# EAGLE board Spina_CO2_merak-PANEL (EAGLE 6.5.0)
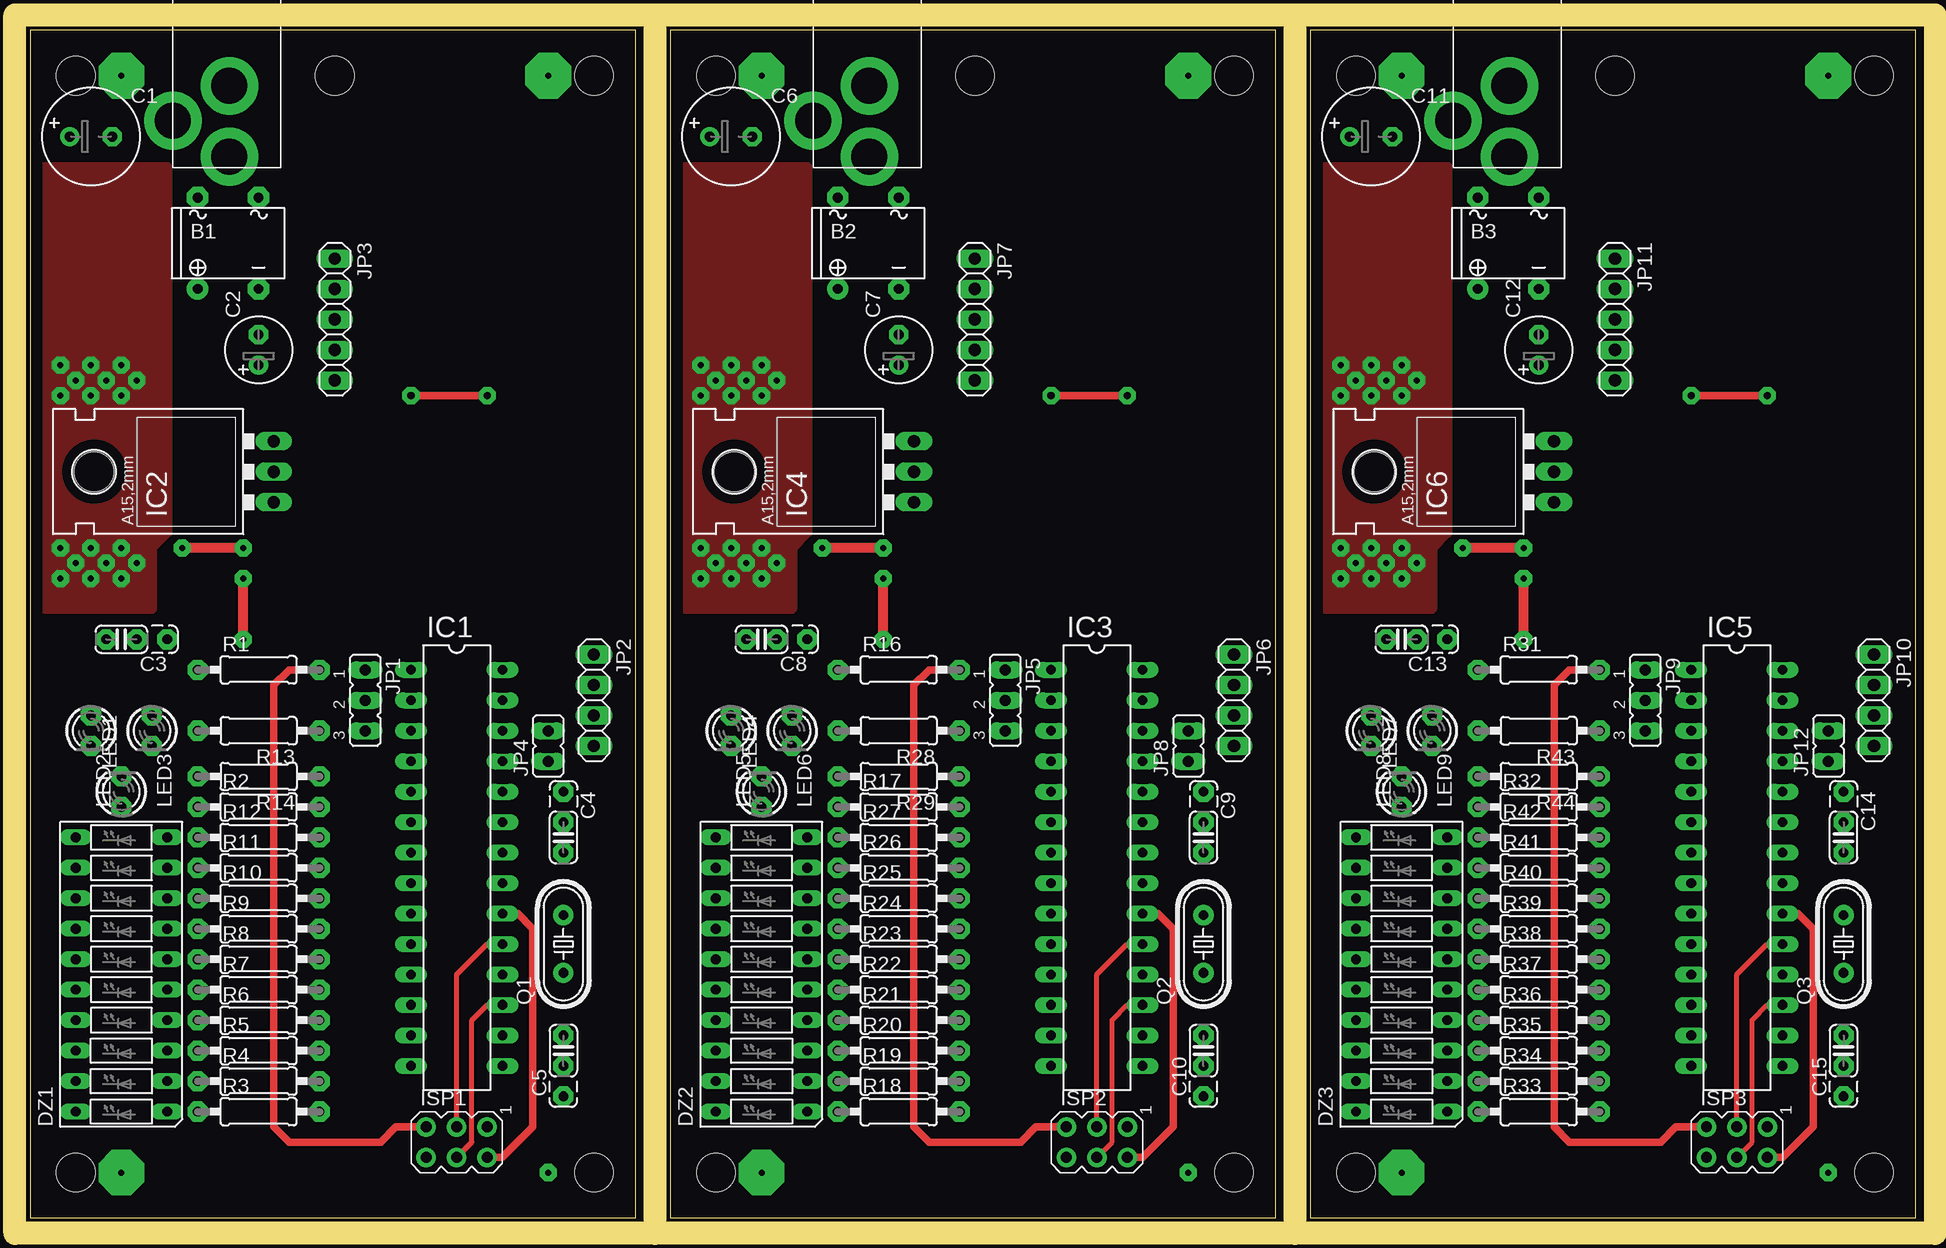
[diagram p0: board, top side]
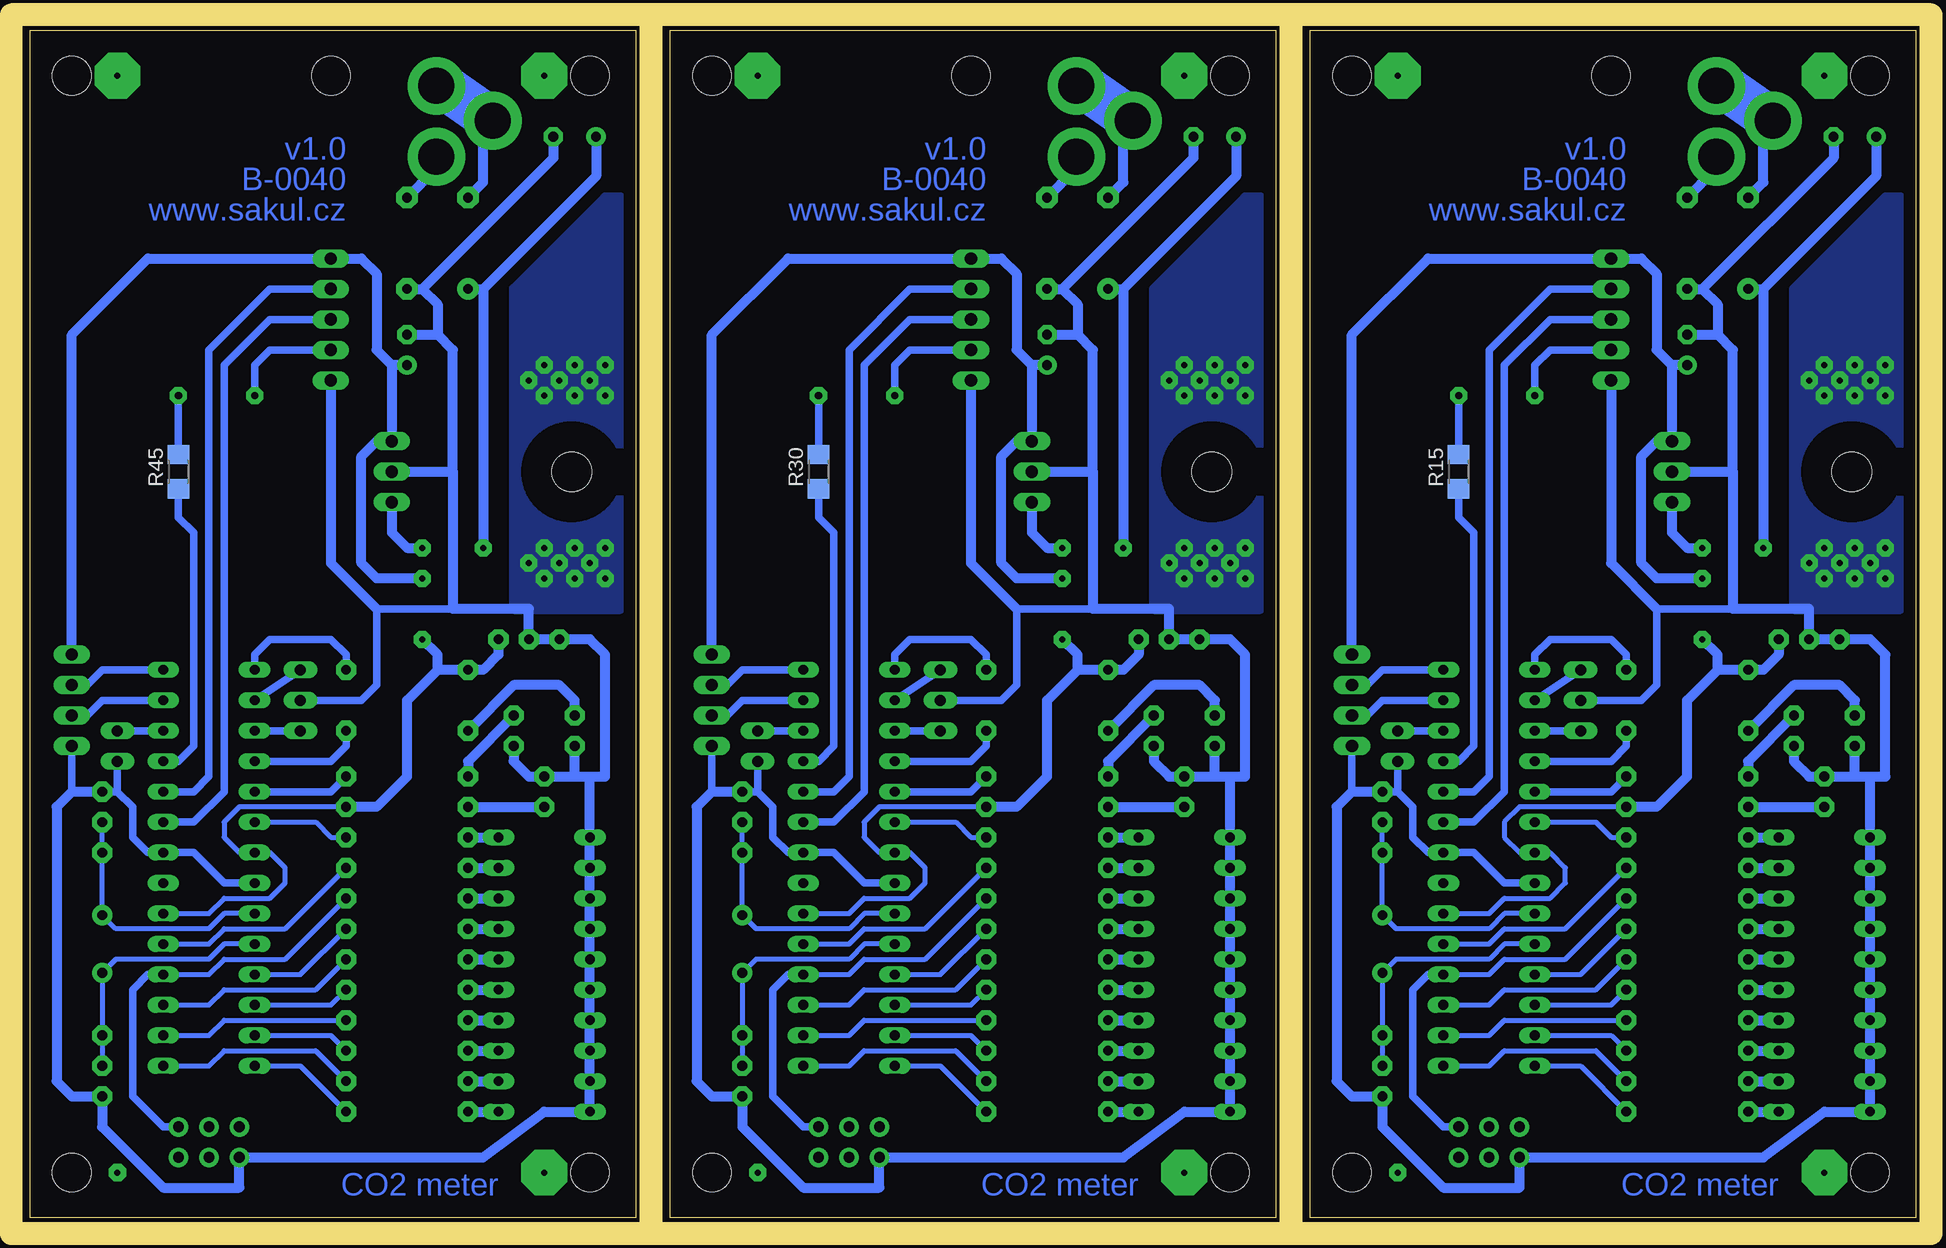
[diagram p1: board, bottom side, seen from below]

Size 157.15 x 99.04 mm. Coordinates in mm from the lower left corner, seen from the top.
Outline: 0,99.04 0,0 50.47,0 50.47,99.04 0,99.04
Outline: 53.34,99.04 53.34,0 103.81,0 103.81,99.04 53.34,99.04
Outline: 106.68,99.04 106.68,0 157.15,0 157.15,99.04 106.68,99.04
Copper layers (1*16): Top 0.035mm / dielectric 1.5mm / Bottom 0.035mm
Design rules "default": minimum track width 10mil, minimum drill 24mil, track to track 8mil, track to pad 8mil, pad to pad 8mil, via to via 8mil, smd to smd 8mil, copper to edge 40mil, drill to drill 8mil, minimum pad ring 10mil, minimum via ring 8mil, stop-mask expansion 4mil, vias tented up to drill 0mil, thermal gap 10mil
Holes 3.2 mm at 3.81,95.23 3.81,3.79 46.99,3.79 46.99,95.23 25.4,95.23 57.15,95.23 57.15,3.79 100.33,3.79 100.33,95.23 78.74,95.23 110.49,95.23 110.49,3.79 153.67,3.79 153.67,95.23 132.08,95.23
Milling: 10 lines

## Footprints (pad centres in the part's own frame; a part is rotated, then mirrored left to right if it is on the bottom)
B-DIL = drill 0.813 pad 1.778: + -2.54,-3.81 | drill 0.813 pad 1.778 octagon: - 2.54,-3.81; AC1 2.54,3.81; AC2 -2.54,3.81
E3,5-8 = drill 0.813 pad 1.6: + -1.778,0 | drill 0.813 pad 1.6 octagon: - 1.778,0
E2,5-6 = drill 0.813 pad 1.6: + -1.27,0 | drill 0.813 pad 1.6 octagon: - 1.27,0
C025_050-024X070 = drill 0.813 pad 1.676 octagon: 1 -3.81,0; 2 -1.27,0; 3 1.27,0
LB10 = drill 0.813 long: 1 -11.43,-3.81; 2 -8.89,-3.81; 3 -6.35,-3.81; 4 -3.81,-3.81; 5 -1.27,-3.81; 6 1.27,-3.81; 7 3.81,-3.81; 8 6.35,-3.81; 9 8.89,-3.81; 10 11.43,-3.81; 11 11.43,3.81; 12 8.89,3.81; 13 6.35,3.81; 14 3.81,3.81; 15 1.27,3.81; 16 -1.27,3.81; 17 -3.81,3.81; 18 -6.35,3.81; 19 -8.89,3.81; 20 -11.43,3.81
DIL28-3 = drill 0.813 long: 1 -16.51,-3.81; 2 -13.97,-3.81; 3 -11.43,-3.81; 4 -8.89,-3.81; 5 -6.35,-3.81; 6 -3.81,-3.81; 7 -1.27,-3.81; 8 1.27,-3.81; 9 3.81,-3.81; 10 6.35,-3.81; 11 8.89,-3.81; 12 11.43,-3.81; 13 13.97,-3.81; 14 16.51,-3.81; 15 16.51,3.81; 16 13.97,3.81; 17 11.43,3.81; 18 8.89,3.81; 19 6.35,3.81; 20 3.81,3.81; 21 1.27,3.81; 22 -1.27,3.81; 23 -3.81,3.81; 24 -6.35,3.81; 25 -8.89,3.81; 26 -11.43,3.81; 27 -13.97,3.81; 28 -16.51,3.81
78XXL = drill 1.016 long: GND 0,-3.81; IN -2.54,-3.81; OUT 2.54,-3.81 | hole 3.302: 0,11.176
AVRISP = drill 0.9 pad 1.626: 1 -1.27,2.54; 2 1.27,2.54; 3 -1.27,0; 4 1.27,0; 5 -1.27,-2.54; 6 1.27,-2.54
JP2 = drill 0.914 long: 1 -2.54,0; 2 0,0; 3 2.54,0
1X04 = drill 1.016 long: 1 -3.81,0; 2 -1.27,0; 3 1.27,0; 4 3.81,0
1X05 = drill 1.016 long: 1 -5.08,0; 2 -2.54,0; 3 0,0; 4 2.54,0; 5 5.08,0
JP1 = drill 0.914 long: 1 0,-1.27; 2 0,1.27
LED3MM = drill 0.813 pad 1.676 octagon: A -1.27,0; K 1.27,0
HC49/S = drill 0.813 pad 1.676: 1 -2.413,0; 2 2.413,0
0207/10 = drill 0.813 pad 1.676 octagon: 1 -5.08,0; 2 5.08,0
R1206 = smd 1.6 x 1.803: 1 -1.422,0; 2 1.422,0
PJ-102A = drill 3 pad 4.8: RING 0.1,-3.39; RING_SW -4.6,-6.29; TIP 0.1,-9.29

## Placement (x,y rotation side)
B1  [B-DIL]  16.51,81.26 0 top
B2  [B-DIL]  69.85,81.26 0 top
B3  [B-DIL]  123.19,81.26 0 top
C1  470uF/25V  [E3,5-8]  5.08,90.15 0 top
C2  100uF/10V  [E2,5-6]  19.05,72.37 90 top
C3  100nF  [C025_050-024X070]  7.62,48.24 180 top
C4  22pF  [C025_050-024X070]  44.45,31.73 270 top
C5  22pF  [C025_050-024X070]  44.45,13.95 90 top
C6  470uF/25V  [E3,5-8]  58.42,90.15 0 top
C7  100uF/10V  [E2,5-6]  72.39,72.37 90 top
C8  100nF  [C025_050-024X070]  60.96,48.24 180 top
C9  22pF  [C025_050-024X070]  97.79,31.73 270 top
C10  22pF  [C025_050-024X070]  97.79,13.95 90 top
C11  470uF/25V  [E3,5-8]  111.76,90.15 0 top
C12  100uF/10V  [E2,5-6]  125.73,72.37 90 top
C13  100nF  [C025_050-024X070]  114.3,48.24 180 top
C14  22pF  [C025_050-024X070]  151.13,31.73 270 top
C15  22pF  [C025_050-024X070]  151.13,13.95 90 top
DZ1  LB10  [LB10]  7.62,20.3 90 top
DZ2  LB10  [LB10]  60.96,20.3 90 top
DZ3  LB10  [LB10]  114.3,20.3 90 top
IC1  ATMEGA8-PU  [DIL28-3]  35.56,29.19 270 top
IC2  7805  [78XXL]  16.51,62.21 90 top
IC3  ATMEGA8-PU  [DIL28-3]  88.9,29.19 270 top
IC4  7805  [78XXL]  69.85,62.21 90 top
IC5  ATMEGA8-PU  [DIL28-3]  142.24,29.19 270 top
IC6  7805  [78XXL]  123.19,62.21 90 top
ISP1  AVRISP-6  [AVRISP]  35.56,6.33 270 top
ISP2  AVRISP-6  [AVRISP]  88.9,6.33 270 top
ISP3  AVRISP-6  [AVRISP]  142.24,6.33 270 top
JP1  [JP2]  27.94,43.16 270 top
JP2  [1X04]  46.99,43.16 270 top
JP3  [1X05]  25.4,74.91 270 top
JP4  [JP1]  43.18,39.35 0 top
JP5  [JP2]  81.28,43.16 270 top
JP6  [1X04]  100.33,43.16 270 top
JP7  [1X05]  78.74,74.91 270 top
JP8  [JP1]  96.52,39.35 0 top
JP9  [JP2]  134.62,43.16 270 top
JP10  [1X04]  153.67,43.16 270 top
JP11  [1X05]  132.08,74.91 270 top
JP12  [JP1]  149.86,39.35 0 top
LED1  [LED3MM]  7.62,35.54 90 top
LED2  [LED3MM]  5.08,40.62 270 top
LED3  [LED3MM]  10.16,40.62 270 top
LED4  [LED3MM]  60.96,35.54 90 top
LED5  [LED3MM]  58.42,40.62 270 top
LED6  [LED3MM]  63.5,40.62 270 top
LED7  [LED3MM]  114.3,35.54 90 top
LED8  [LED3MM]  111.76,40.62 270 top
LED9  [LED3MM]  116.84,40.62 270 top
Q1  16MHz  [HC49/S]  44.45,22.84 90 top
Q2  16MHz  [HC49/S]  97.79,22.84 90 top
Q3  16MHz  [HC49/S]  151.13,22.84 90 top
R1  12K  [0207/10]  19.05,45.7 0 top
R2  1K  [0207/10]  19.05,34.27 0 top
R3  1K  [0207/10]  19.05,8.87 0 top
R4  1K  [0207/10]  19.05,11.41 0 top
R5  1K  [0207/10]  19.05,13.95 0 top
R6  1K  [0207/10]  19.05,16.49 0 top
R7  1K  [0207/10]  19.05,19.03 0 top
R8  1K  [0207/10]  19.05,21.57 0 top
R9  1K  [0207/10]  19.05,24.11 0 top
R10  1K  [0207/10]  19.05,26.65 0 top
R11  1K  [0207/10]  19.05,29.19 0 top
R12  1K  [0207/10]  19.05,31.73 0 top
R13  1K  [0207/10]  19.05,40.62 180 top
R14  1K  [0207/10]  19.05,36.81 180 top
R15  NONE/0R  [R1206]  38.1,62.21 90 bottom
R16  12K  [0207/10]  72.39,45.7 0 top
R17  1K  [0207/10]  72.39,34.27 0 top
R18  1K  [0207/10]  72.39,8.87 0 top
R19  1K  [0207/10]  72.39,11.41 0 top
R20  1K  [0207/10]  72.39,13.95 0 top
R21  1K  [0207/10]  72.39,16.49 0 top
R22  1K  [0207/10]  72.39,19.03 0 top
R23  1K  [0207/10]  72.39,21.57 0 top
R24  1K  [0207/10]  72.39,24.11 0 top
R25  1K  [0207/10]  72.39,26.65 0 top
R26  1K  [0207/10]  72.39,29.19 0 top
R27  1K  [0207/10]  72.39,31.73 0 top
R28  1K  [0207/10]  72.39,40.62 180 top
R29  1K  [0207/10]  72.39,36.81 180 top
R30  NONE/0R  [R1206]  91.44,62.21 90 bottom
R31  12K  [0207/10]  125.73,45.7 0 top
R32  1K  [0207/10]  125.73,34.27 0 top
R33  1K  [0207/10]  125.73,8.87 0 top
R34  1K  [0207/10]  125.73,11.41 0 top
R35  1K  [0207/10]  125.73,13.95 0 top
R36  1K  [0207/10]  125.73,16.49 0 top
R37  1K  [0207/10]  125.73,19.03 0 top
R38  1K  [0207/10]  125.73,21.57 0 top
R39  1K  [0207/10]  125.73,24.11 0 top
R40  1K  [0207/10]  125.73,26.65 0 top
R41  1K  [0207/10]  125.73,29.19 0 top
R42  1K  [0207/10]  125.73,31.73 0 top
R43  1K  [0207/10]  125.73,40.62 180 top
R44  1K  [0207/10]  125.73,36.81 180 top
R45  NONE/0R  [R1206]  144.78,62.21 90 bottom
U$1  2.1MMJACKTHM  [PJ-102A]  16.51,97.77 0 top
U$2  2.1MMJACKTHM  [PJ-102A]  69.85,97.77 0 top
U$3  2.1MMJACKTHM  [PJ-102A]  123.19,97.77 0 top

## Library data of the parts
B1-B3 = rectifier
C1-C15 R1-R45 = rcl
DZ1-DZ3 LED1-LED9 = led
IC1 IC3 IC5 = atmega8
IC2 IC4 IC6 = v-reg
ISP1-ISP3 U$1-U$3 = adafruit
JP1 JP4 JP5 JP8 JP9 JP12 = jumper
JP2 JP3 JP6 JP7 JP10 JP11 = pinhead
Q1-Q3 = crystal; OC_FARNELL: 1667008; OC_NEWARK: unknown

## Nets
+5V: C2.+ C3.1 IC1.7 IC1.20 IC2.OUT ISP1.2 JP2.1 JP3.1 R1.1 R2.2
+5V1: C7.+ C8.1 IC3.7 IC3.20 IC4.OUT ISP2.2 JP6.1 JP7.1 R16.1 R17.2
+5V2: C12.+ C13.1 IC5.7 IC5.20 IC6.OUT ISP3.2 JP10.1 JP11.1 R31.1 R32.2
GND: B1.- C1.- C2.- C3.2 C4.1 C5.1 DZ1.11 DZ1.12 DZ1.13 DZ1.14 DZ1.15 DZ1.16 DZ1.17 DZ1.18 DZ1.19 DZ1.20 IC1.8 IC1.22 IC2.GND ISP1.6 JP1.2 JP2.4 JP3.5 JP4.1 LED1.K LED2.K LED3.K
GND1: B2.- C6.- C7.- C8.2 C9.1 C10.1 DZ2.11 DZ2.12 DZ2.13 DZ2.14 DZ2.15 DZ2.16 DZ2.17 DZ2.18 DZ2.19 DZ2.20 IC3.8 IC3.22 IC4.GND ISP2.6 JP5.2 JP6.4 JP7.5 JP8.1 LED4.K LED5.K LED6.K
GND2: B3.- C11.- C12.- C13.2 C14.1 C15.1 DZ3.11 DZ3.12 DZ3.13 DZ3.14 DZ3.15 DZ3.16 DZ3.17 DZ3.18 DZ3.19 DZ3.20 IC5.8 IC5.22 IC6.GND ISP3.6 JP9.2 JP10.4 JP11.5 JP12.1 LED7.K LED8.K LED9.K
MISO: IC1.18 ISP1.1 R10.2
MISO1: IC3.18 ISP2.1 R25.2
MISO2: IC5.18 ISP3.1 R40.2
MOSI: IC1.17 ISP1.4 R8.2
MOSI1: IC3.17 ISP2.4 R23.2
MOSI2: IC5.17 ISP3.4 R38.2
N$1: B1.AC1 U$1.TIP
N$2: B1.AC2 U$1.RING U$1.RING_SW
N$3: B1.+ C1.+ IC2.IN
N$4: C4.2 IC1.9 Q1.2
N$5: C5.2 IC1.10 Q1.1
N$6: DZ1.5 R7.1
N$7: IC1.1 ISP1.5 R1.2
N$8: DZ1.10 R12.1
N$9: LED1.A R2.1
N$10: IC1.2 JP1.1
N$11: IC1.3 JP1.3
N$12: DZ1.9 R11.1
N$13: DZ1.8 R10.1
N$14: DZ1.7 R9.1
N$15: DZ1.2 R4.1
N$16: DZ1.3 R5.1
N$17: DZ1.4 R6.1
N$18: DZ1.6 R8.1
N$19: DZ1.1 R3.1
N$20: IC1.24 JP3.2
N$21: IC1.23 JP3.3
N$22: IC1.25 R15.1
N$23: IC1.16 R6.2
N$24: IC1.14 R3.2
N$25: IC1.15 R4.2
N$26: IC1.13 R5.2
N$27: IC1.11 R9.2
N$28: IC1.12 R7.2
N$29: IC1.6 R12.2
N$30: JP3.4 R15.2
N$31: IC1.26 JP4.2
N$33: LED2.A R13.2
N$34: LED3.A R14.2
N$35: IC1.4 R13.1
N$36: IC1.5 R14.1
N$40: B2.AC1 U$2.TIP
N$41: B2.AC2 U$2.RING U$2.RING_SW
N$42: B2.+ C6.+ IC4.IN
N$43: C9.2 IC3.9 Q2.2
N$44: C10.2 IC3.10 Q2.1
N$45: IC3.1 ISP2.5 R16.2
N$46: LED4.A R17.1
N$47: IC3.2 JP5.1
N$48: IC3.3 JP5.3
N$49: DZ2.5 R22.1
N$50: DZ2.10 R27.1
N$51: DZ2.9 R26.1
N$52: DZ2.8 R25.1
N$53: DZ2.7 R24.1
N$54: DZ2.2 R19.1
N$55: DZ2.3 R20.1
N$56: DZ2.4 R21.1
N$57: DZ2.6 R23.1
N$58: DZ2.1 R18.1
N$59: IC3.16 R21.2
N$60: LED5.A R28.2
N$61: LED6.A R29.2
N$62: IC3.4 R28.1
N$63: IC3.5 R29.1
N$64: IC3.24 JP7.2
N$65: IC3.23 JP7.3
N$66: IC3.25 R30.1
N$67: JP7.4 R30.2
N$68: IC3.26 JP8.2
N$71: IC3.14 R18.2
N$72: IC3.15 R19.2
N$73: IC3.13 R20.2
N$74: IC3.11 R24.2
N$75: IC3.12 R22.2
N$76: IC3.6 R27.2
N$79: B3.AC1 U$3.TIP
N$80: B3.AC2 U$3.RING U$3.RING_SW
N$81: B3.+ C11.+ IC6.IN
N$82: C14.2 IC5.9 Q3.2
N$83: C15.2 IC5.10 Q3.1
N$84: IC5.1 ISP3.5 R31.2
N$85: LED7.A R32.1
N$86: IC5.2 JP9.1
N$87: IC5.3 JP9.3
N$88: DZ3.5 R37.1
N$89: DZ3.10 R42.1
N$90: DZ3.9 R41.1
N$91: DZ3.8 R40.1
N$92: DZ3.7 R39.1
N$93: DZ3.2 R34.1
N$94: DZ3.3 R35.1
N$95: DZ3.4 R36.1
N$96: DZ3.6 R38.1
N$97: DZ3.1 R33.1
N$98: IC5.16 R36.2
N$99: LED8.A R43.2
N$100: LED9.A R44.2
N$101: IC5.4 R43.1
N$102: IC5.5 R44.1
N$103: IC5.24 JP11.2
N$104: IC5.23 JP11.3
N$105: IC5.25 R45.1
N$106: JP11.4 R45.2
N$107: IC5.26 JP12.2
N$110: IC5.14 R33.2
N$111: IC5.15 R34.2
N$112: IC5.13 R35.2
N$113: IC5.11 R39.2
N$114: IC5.12 R37.2
N$115: IC5.6 R42.2
SCK: IC1.19 ISP1.3 R11.2
SCK1: IC3.19 ISP2.3 R26.2
SCK2: IC5.19 ISP3.3 R41.2
SCL: IC1.28 JP2.2
SCL1: IC3.28 JP6.2
SCL2: IC5.28 JP10.2
SDA: IC1.27 JP2.3
SDA1: IC3.27 JP6.3
SDA2: IC5.27 JP10.3

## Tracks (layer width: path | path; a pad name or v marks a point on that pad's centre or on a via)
+5V  (via drill 0.5 pad 1.42)
  Top 0.61: ISP1.2 39.37,5.06 41.91,7.6 41.91,24.11 40.64,25.38 IC1.20
  Top 0.813: v17.78,48.24 v17.78,53.32
  Bottom 0.406: IC1.20 35.56,25.38 34.29,26.65 30.48,26.65 29.21,27.92 29.21,29.19 30.48,30.46 IC1.7 33.02,30.46 34.29,31.73 34.29,33 33.02,34.27 21.59,34.27
  Bottom 0.813: R2.2 21.59,34.27 19.05,36.81 19.05,43.16 16.51,45.7 | JP2.1 46.99,73.64 40.64,79.99 JP3.1 22.86,79.99 21.59,78.72 21.59,72.37 20.32,71.1 | C2.+ 20.32,71.1 | 20.32,71.1 IC2.OUT 21.59,64.75 22.86,63.48 22.86,54.59 21.59,53.32 v17.78,53.32 | C3.1 11.43,46.97 12.7,45.7 R1.1 16.51,45.7 | 16.51,45.7 16.51,46.97 v17.78,48.24
+5V1  (via drill 0.5 pad 1.42)
  Top 0.61: ISP2.2 92.71,5.06 95.25,7.6 95.25,24.11 93.98,25.38 IC3.20
  Top 0.813: v71.12,48.24 v71.12,53.32
  Bottom 0.406: IC3.20 88.9,25.38 87.63,26.65 83.82,26.65 82.55,27.92 82.55,29.19 83.82,30.46 IC3.7 86.36,30.46 87.63,31.73 87.63,33 86.36,34.27 74.93,34.27
  Bottom 0.813: R17.2 74.93,34.27 72.39,36.81 72.39,43.16 69.85,45.7 | JP6.1 100.33,73.64 93.98,79.99 JP7.1 76.2,79.99 74.93,78.72 74.93,72.37 73.66,71.1 | C7.+ 73.66,71.1 | 73.66,71.1 IC4.OUT 74.93,64.75 76.2,63.48 76.2,54.59 74.93,53.32 v71.12,53.32 | C8.1 64.77,46.97 66.04,45.7 R16.1 69.85,45.7 | 69.85,45.7 69.85,46.97 v71.12,48.24
+5V2  (via drill 0.5 pad 1.42)
  Top 0.61: ISP3.2 146.05,5.06 148.59,7.6 148.59,24.11 147.32,25.38 IC5.20
  Top 0.813: v124.46,48.24 v124.46,53.32
  Bottom 0.406: IC5.20 142.24,25.38 140.97,26.65 137.16,26.65 135.89,27.92 135.89,29.19 137.16,30.46 IC5.7 139.7,30.46 140.97,31.73 140.97,33 139.7,34.27 128.27,34.27
  Bottom 0.813: R32.2 128.27,34.27 125.73,36.81 125.73,43.16 123.19,45.7 | JP10.1 153.67,73.64 147.32,79.99 JP11.1 129.54,79.99 128.27,78.72 128.27,72.37 127,71.1 | C12.+ 127,71.1 | 127,71.1 IC6.OUT 128.27,64.75 129.54,63.48 129.54,54.59 128.27,53.32 v124.46,53.32 | C13.1 118.11,46.97 119.38,45.7 R31.1 123.19,45.7 | 123.19,45.7 123.19,46.97 v124.46,48.24
GND  (via drill 0.5 pad 1.42)
  Bottom 0.61: 43.18,35.54 41.91,34.27 41.91,31.73 40.64,30.46 IC1.22 36.83,30.46 34.29,27.92 IC1.8 | 43.18,35.54 C4.1 | JP4.1 43.18,35.54 | JP2.4 46.99,35.54 | JP1.2 22.86,43.16 21.59,44.43 21.59,50.78 15.24,50.78
  Bottom 0.813: 3.81,36.81 DZ1.11 DZ1.12 DZ1.13 DZ1.14 DZ1.15 DZ1.16 DZ1.17 DZ1.18 DZ1.19 DZ1.20 7.62,8.87 12.7,5.06 ISP1.6 33.02,2.52 39.37,2.52 44.45,7.6 C5.1 46.99,10.14 48.26,11.41 48.26,34.27 46.99,35.54 C4.1 | 5.08,36.81 LED2.K | 5.08,36.81 LED1.K 8.89,36.81 10.16,38.08 LED3.K | 5.08,36.81 3.81,36.81 | 3.81,36.81 2.54,36.81 2.54,46.97 3.81,48.24 C3.2 8.89,50.78 15.24,50.78 15.24,62.21 | C1.- 6.86,88.37 17.78,77.45 | B1.- 17.78,77.45 | 17.78,77.45 16.51,76.18 16.51,73.64 | IC2.GND 15.24,62.21 | 15.24,62.21 15.24,72.37 16.51,73.64 | C2.- 16.51,73.64 | JP3.5 25.4,54.59 21.59,50.78
  other vias: 8.89,69.83 7.62,71.1 7.62,68.56 6.35,69.83 5.08,71.1 5.08,68.56 3.81,69.83 2.54,68.56 2.54,71.1 8.89,54.59 7.62,55.86 7.62,53.32 6.35,54.59 5.08,53.32 5.08,55.86 3.81,54.59 2.54,53.32 2.54,55.86
  pour Bottom: 1.27,85.07 2.54,85.07 10.16,77.45 10.16,50.78 1.27,50.78
  pour Top: 11.43,87.61 11.43,57.13 10.16,55.86 10.16,50.78 1.27,50.78 1.27,87.61
GND1  (via drill 0.5 pad 1.42)
  Bottom 0.61: 96.52,35.54 95.25,34.27 95.25,31.73 93.98,30.46 IC3.22 90.17,30.46 87.63,27.92 IC3.8 | 96.52,35.54 C9.1 | JP8.1 96.52,35.54 | JP6.4 100.33,35.54 | JP5.2 76.2,43.16 74.93,44.43 74.93,50.78 68.58,50.78
  Bottom 0.813: 57.15,36.81 DZ2.11 DZ2.12 DZ2.13 DZ2.14 DZ2.15 DZ2.16 DZ2.17 DZ2.18 DZ2.19 DZ2.20 60.96,8.87 66.04,5.06 ISP2.6 86.36,2.52 92.71,2.52 97.79,7.6 C10.1 100.33,10.14 101.6,11.41 101.6,34.27 100.33,35.54 C9.1 | 58.42,36.81 LED5.K | 58.42,36.81 LED4.K 62.23,36.81 63.5,38.08 LED6.K | 58.42,36.81 57.15,36.81 | 57.15,36.81 55.88,36.81 55.88,46.97 57.15,48.24 C8.2 62.23,50.78 68.58,50.78 68.58,62.21 | C6.- 60.2,88.37 71.12,77.45 | B2.- 71.12,77.45 | 71.12,77.45 69.85,76.18 69.85,73.64 | IC4.GND 68.58,62.21 | 68.58,62.21 68.58,72.37 69.85,73.64 | C7.- 69.85,73.64 | JP7.5 78.74,54.59 74.93,50.78
  other vias: 62.23,69.83 60.96,71.1 60.96,68.56 59.69,69.83 58.42,71.1 58.42,68.56 57.15,69.83 55.88,68.56 55.88,71.1 62.23,54.59 60.96,55.86 60.96,53.32 59.69,54.59 58.42,53.32 58.42,55.86 57.15,54.59 55.88,53.32 55.88,55.86
  pour Bottom: 54.61,85.07 55.88,85.07 63.5,77.45 63.5,50.78 54.61,50.78
  pour Top: 64.77,87.61 64.77,57.13 63.5,55.86 63.5,50.78 54.61,50.78 54.61,87.61
GND2  (via drill 0.5 pad 1.42)
  Bottom 0.61: 149.86,35.54 148.59,34.27 148.59,31.73 147.32,30.46 IC5.22 143.51,30.46 140.97,27.92 IC5.8 | 149.86,35.54 C14.1 | JP12.1 149.86,35.54 | JP10.4 153.67,35.54 | JP9.2 129.54,43.16 128.27,44.43 128.27,50.78 121.92,50.78
  Bottom 0.813: 110.49,36.81 DZ3.11 DZ3.12 DZ3.13 DZ3.14 DZ3.15 DZ3.16 DZ3.17 DZ3.18 DZ3.19 DZ3.20 114.3,8.87 119.38,5.06 ISP3.6 139.7,2.52 146.05,2.52 151.13,7.6 C15.1 153.67,10.14 154.94,11.41 154.94,34.27 153.67,35.54 C14.1 | 111.76,36.81 LED8.K | 111.76,36.81 LED7.K 115.57,36.81 116.84,38.08 LED9.K | 111.76,36.81 110.49,36.81 | 110.49,36.81 109.22,36.81 109.22,46.97 110.49,48.24 C13.2 115.57,50.78 121.92,50.78 121.92,62.21 | C11.- 113.54,88.37 124.46,77.45 | B3.- 124.46,77.45 | 124.46,77.45 123.19,76.18 123.19,73.64 | IC6.GND 121.92,62.21 | 121.92,62.21 121.92,72.37 123.19,73.64 | C12.- 123.19,73.64 | JP11.5 132.08,54.59 128.27,50.78
  other vias: 115.57,69.83 114.3,71.1 114.3,68.56 113.03,69.83 111.76,71.1 111.76,68.56 110.49,69.83 109.22,68.56 109.22,71.1 115.57,54.59 114.3,55.86 114.3,53.32 113.03,54.59 111.76,53.32 111.76,55.86 110.49,54.59 109.22,53.32 109.22,55.86
  pour Bottom: 107.95,85.07 109.22,85.07 116.84,77.45 116.84,50.78 107.95,50.78
  pour Top: 118.11,87.61 118.11,57.13 116.84,55.86 116.84,50.78 107.95,50.78 107.95,87.61
MISO
  Bottom 0.406: IC1.18 35.56,20.3 34.29,21.57 29.21,21.57 R10.2
  Bottom 0.61: ISP1.1 39.37,7.6 41.91,10.14 41.91,19.03 40.64,20.3 IC1.18
MISO1
  Bottom 0.406: IC3.18 88.9,20.3 87.63,21.57 82.55,21.57 R25.2
  Bottom 0.61: ISP2.1 92.71,7.6 95.25,10.14 95.25,19.03 93.98,20.3 IC3.18
MISO2
  Bottom 0.406: IC5.18 142.24,20.3 140.97,21.57 135.89,21.57 R40.2
  Bottom 0.61: ISP3.1 146.05,7.6 148.59,10.14 148.59,19.03 147.32,20.3 IC5.18
MOSI
  Top 0.406: ISP1.4 36.83,6.33 36.83,16.49 38.1,17.76 IC1.17
  Bottom 0.406: IC1.17 35.56,17.76 34.29,19.03 26.67,19.03 R8.2
MOSI1
  Top 0.406: ISP2.4 90.17,6.33 90.17,16.49 91.44,17.76 IC3.17
  Bottom 0.406: IC3.17 88.9,17.76 87.63,19.03 80.01,19.03 R23.2
MOSI2
  Top 0.406: ISP3.4 143.51,6.33 143.51,16.49 144.78,17.76 IC5.17
  Bottom 0.406: IC5.17 142.24,17.76 140.97,19.03 133.35,19.03 R38.2
N$1
  Bottom 0.813: U$1.TIP 17.88,86.24 B1.AC1
N$2
  Bottom 0.813: B1.AC2 12.7,86.34 12.7,91 U$1.RING_SW
  Bottom 3.81: U$1.RING 16.08,94.38 U$1.RING_SW
N$3  (via drill 0.5 pad 1.42)
  Top 0.813: v17.78,55.86 v12.7,55.86
  Bottom 0.813: C1.+ 3.3,86.85 12.7,77.45 | IC2.IN 20.32,57.13 19.05,55.86 v17.78,55.86 | B1.+ 12.7,77.45 | 12.7,77.45 v12.7,55.86
N$4
  Bottom 0.406: C4.2 Q1.2 43.31,24.11 35.56,24.11 34.29,25.38 IC1.9
N$5
  Bottom 0.406: IC1.10 34.29,22.84 35.56,21.57 43.31,21.57 Q1.1 C5.2
N$6
  Bottom 0.813: R7.1 DZ1.5
N$7
  Top 0.61: R1.2 21.59,45.7 20.32,44.43 20.32,7.6 21.59,6.33 29.21,6.33 30.48,7.6 ISP1.5
  Bottom 0.61: IC1.1 31.75,46.97 30.48,48.24 25.4,48.24 24.13,46.97 R1.2
N$8
  Bottom 0.813: R12.1 DZ1.10
N$9
  Bottom 0.813: R2.1 LED1.A
N$10
  Bottom 0.61: IC1.2 JP1.1
N$11
  Bottom 0.61: IC1.3 JP1.3
N$12
  Bottom 0.813: R11.1 DZ1.9
N$13
  Bottom 0.813: R10.1 DZ1.8
N$14
  Bottom 0.813: R9.1 DZ1.7
N$15
  Bottom 0.813: R4.1 DZ1.2
N$16
  Bottom 0.813: R5.1 DZ1.3
N$17
  Bottom 0.813: R6.1 DZ1.4
N$18
  Bottom 0.813: R8.1 DZ1.6
N$19
  Bottom 0.813: R3.1 DZ1.1
N$20
  Bottom 0.61: IC1.24 36.83,35.54 35.56,36.81 35.56,72.37 30.48,77.45 JP3.2
N$21
  Bottom 0.61: IC1.23 36.83,33 34.29,35.54 34.29,71.1 30.48,74.91 JP3.3
N$22
  Bottom 0.61: IC1.25 38.1,38.08 36.83,39.35 36.83,57.13 38.1,58.4 R15.1
N$23
  Bottom 0.406: IC1.16 35.56,15.22 34.29,16.49 R6.2
N$24
  Bottom 0.406: IC1.14 27.94,12.68 R3.2
N$25
  Bottom 0.406: IC1.15 35.56,12.68 34.29,13.95 26.67,13.95 R4.2
N$26
  Bottom 0.406: IC1.13 25.4,15.22 R5.2
N$27
  Bottom 0.406: IC1.11 27.94,20.3 R9.2
N$28
  Bottom 0.406: IC1.12 25.4,17.76 R7.2
N$29
  Bottom 0.406: IC1.6 26.67,33 25.4,31.73 R12.2
N$30  (via drill 0.6 pad 1.42)
  Top 0.61: v38.1,68.56 v31.75,68.56
  Bottom 0.61: R15.2 v38.1,68.56 | JP3.4 30.48,72.37 31.75,71.1 v31.75,68.56
N$31
  Bottom 0.61: IC1.26 JP4.2
N$32  (via drill 0.5 pad 3.81)
  other vias: 7.62,95.23
N$33
  Bottom 0.813: LED2.A 5.08,43.16 6.35,44.43 10.16,44.43 R13.2
N$34
  Bottom 0.813: LED3.A 13.97,38.08 R14.2
N$35
  Bottom 0.61: IC1.4 25.4,38.08 24.13,39.35 R13.1
N$36
  Bottom 0.61: R14.1 25.4,35.54 IC1.5
N$37  (via drill 0.5 pad 3.81)
  other vias: 7.62,3.79
N$38  (via drill 0.5 pad 3.81)
  other vias: 43.18,95.23
N$39  (via drill 0.5 pad 1.42)
  other vias: 43.18,3.79
N$40
  Bottom 0.813: U$2.TIP 71.22,86.24 B2.AC1
N$41
  Bottom 0.813: B2.AC2 66.04,86.34 66.04,91 U$2.RING_SW
  Bottom 3.81: U$2.RING 69.42,94.38 U$2.RING_SW
N$42  (via drill 0.5 pad 1.42)
  Top 0.813: v71.12,55.86 v66.04,55.86
  Bottom 0.813: C6.+ 56.64,86.85 66.04,77.45 | IC4.IN 73.66,57.13 72.39,55.86 v71.12,55.86 | B2.+ 66.04,77.45 | 66.04,77.45 v66.04,55.86
N$43
  Bottom 0.406: C9.2 Q2.2 96.65,24.11 88.9,24.11 87.63,25.38 IC3.9
N$44
  Bottom 0.406: IC3.10 87.63,22.84 88.9,21.57 96.65,21.57 Q2.1 C10.2
N$45
  Top 0.61: R16.2 74.93,45.7 73.66,44.43 73.66,7.6 74.93,6.33 82.55,6.33 83.82,7.6 ISP2.5
  Bottom 0.61: IC3.1 85.09,46.97 83.82,48.24 78.74,48.24 77.47,46.97 R16.2
N$46
  Bottom 0.813: R17.1 LED4.A
N$47
  Bottom 0.61: IC3.2 JP5.1
N$48
  Bottom 0.61: IC3.3 JP5.3
N$49
  Bottom 0.813: R22.1 DZ2.5
N$50
  Bottom 0.813: R27.1 DZ2.10
N$51
  Bottom 0.813: R26.1 DZ2.9
N$52
  Bottom 0.813: R25.1 DZ2.8
N$53
  Bottom 0.813: R24.1 DZ2.7
N$54
  Bottom 0.813: R19.1 DZ2.2
N$55
  Bottom 0.813: R20.1 DZ2.3
N$56
  Bottom 0.813: R21.1 DZ2.4
N$57
  Bottom 0.813: R23.1 DZ2.6
N$58
  Bottom 0.813: R18.1 DZ2.1
N$59
  Bottom 0.406: IC3.16 88.9,15.22 87.63,16.49 R21.2
N$60
  Bottom 0.813: LED5.A 58.42,43.16 59.69,44.43 63.5,44.43 R28.2
N$61
  Bottom 0.813: LED6.A 67.31,38.08 R29.2
N$62
  Bottom 0.61: IC3.4 78.74,38.08 77.47,39.35 R28.1
N$63
  Bottom 0.61: R29.1 78.74,35.54 IC3.5
N$64
  Bottom 0.61: IC3.24 90.17,35.54 88.9,36.81 88.9,72.37 83.82,77.45 JP7.2
N$65
  Bottom 0.61: IC3.23 90.17,33 87.63,35.54 87.63,71.1 83.82,74.91 JP7.3
N$66
  Bottom 0.61: IC3.25 91.44,38.08 90.17,39.35 90.17,57.13 91.44,58.4 R30.1
N$67  (via drill 0.6 pad 1.42)
  Top 0.61: v91.44,68.56 v85.09,68.56
  Bottom 0.61: R30.2 v91.44,68.56 | JP7.4 83.82,72.37 85.09,71.1 v85.09,68.56
N$68
  Bottom 0.61: IC3.26 JP8.2
N$69  (via drill 0.5 pad 3.81)
  other vias: 60.96,95.23
N$70  (via drill 0.5 pad 3.81)
  other vias: 60.96,3.79
N$71
  Bottom 0.406: IC3.14 81.28,12.68 R18.2
N$72
  Bottom 0.406: IC3.15 88.9,12.68 87.63,13.95 80.01,13.95 R19.2
N$73
  Bottom 0.406: IC3.13 78.74,15.22 R20.2
N$74
  Bottom 0.406: IC3.11 81.28,20.3 R24.2
N$75
  Bottom 0.406: IC3.12 78.74,17.76 R22.2
N$76
  Bottom 0.406: IC3.6 80.01,33 78.74,31.73 R27.2
N$77  (via drill 0.5 pad 3.81)
  other vias: 96.52,95.23
N$78  (via drill 0.5 pad 1.42)
  other vias: 96.52,3.79
N$79
  Bottom 0.813: U$3.TIP 124.56,86.24 B3.AC1
N$80
  Bottom 0.813: B3.AC2 119.38,86.34 119.38,91 U$3.RING_SW
  Bottom 3.81: U$3.RING 122.76,94.38 U$3.RING_SW
N$81  (via drill 0.5 pad 1.42)
  Top 0.813: v124.46,55.86 v119.38,55.86
  Bottom 0.813: C11.+ 109.98,86.85 119.38,77.45 | IC6.IN 127,57.13 125.73,55.86 v124.46,55.86 | B3.+ 119.38,77.45 | 119.38,77.45 v119.38,55.86
N$82
  Bottom 0.406: C14.2 Q3.2 149.99,24.11 142.24,24.11 140.97,25.38 IC5.9
N$83
  Bottom 0.406: IC5.10 140.97,22.84 142.24,21.57 149.99,21.57 Q3.1 C15.2
N$84
  Top 0.61: R31.2 128.27,45.7 127,44.43 127,7.6 128.27,6.33 135.89,6.33 137.16,7.6 ISP3.5
  Bottom 0.61: IC5.1 138.43,46.97 137.16,48.24 132.08,48.24 130.81,46.97 R31.2
N$85
  Bottom 0.813: R32.1 LED7.A
N$86
  Bottom 0.61: IC5.2 JP9.1
N$87
  Bottom 0.61: IC5.3 JP9.3
N$88
  Bottom 0.813: R37.1 DZ3.5
N$89
  Bottom 0.813: R42.1 DZ3.10
N$90
  Bottom 0.813: R41.1 DZ3.9
N$91
  Bottom 0.813: R40.1 DZ3.8
N$92
  Bottom 0.813: R39.1 DZ3.7
N$93
  Bottom 0.813: R34.1 DZ3.2
N$94
  Bottom 0.813: R35.1 DZ3.3
N$95
  Bottom 0.813: R36.1 DZ3.4
N$96
  Bottom 0.813: R38.1 DZ3.6
N$97
  Bottom 0.813: R33.1 DZ3.1
N$98
  Bottom 0.406: IC5.16 142.24,15.22 140.97,16.49 R36.2
N$99
  Bottom 0.813: LED8.A 111.76,43.16 113.03,44.43 116.84,44.43 R43.2
N$100
  Bottom 0.813: LED9.A 120.65,38.08 R44.2
N$101
  Bottom 0.61: IC5.4 132.08,38.08 130.81,39.35 R43.1
N$102
  Bottom 0.61: R44.1 132.08,35.54 IC5.5
N$103
  Bottom 0.61: IC5.24 143.51,35.54 142.24,36.81 142.24,72.37 137.16,77.45 JP11.2
N$104
  Bottom 0.61: IC5.23 143.51,33 140.97,35.54 140.97,71.1 137.16,74.91 JP11.3
N$105
  Bottom 0.61: IC5.25 144.78,38.08 143.51,39.35 143.51,57.13 144.78,58.4 R45.1
N$106  (via drill 0.6 pad 1.42)
  Top 0.61: v144.78,68.56 v138.43,68.56
  Bottom 0.61: R45.2 v144.78,68.56 | JP11.4 137.16,72.37 138.43,71.1 v138.43,68.56
N$107
  Bottom 0.61: IC5.26 JP12.2
N$108  (via drill 0.5 pad 3.81)
  other vias: 114.3,95.23
N$109  (via drill 0.5 pad 3.81)
  other vias: 114.3,3.79
N$110
  Bottom 0.406: IC5.14 134.62,12.68 R33.2
N$111
  Bottom 0.406: IC5.15 142.24,12.68 140.97,13.95 133.35,13.95 R34.2
N$112
  Bottom 0.406: IC5.13 132.08,15.22 R35.2
N$113
  Bottom 0.406: IC5.11 134.62,20.3 R39.2
N$114
  Bottom 0.406: IC5.12 132.08,17.76 R37.2
N$115
  Bottom 0.406: IC5.6 133.35,33 132.08,31.73 R42.2
N$116  (via drill 0.5 pad 3.81)
  other vias: 149.86,95.23
N$117  (via drill 0.5 pad 1.42)
  other vias: 149.86,3.79
SCK
  Top 0.406: ISP1.3 35.56,20.3 38.1,22.84 IC1.19
  Bottom 0.406: IC1.19 35.56,22.84 34.29,24.11 29.21,24.11 R11.2
SCK1
  Top 0.406: ISP2.3 88.9,20.3 91.44,22.84 IC3.19
  Bottom 0.406: IC3.19 88.9,22.84 87.63,24.11 82.55,24.11 R26.2
SCK2
  Top 0.406: ISP3.3 142.24,20.3 144.78,22.84 IC5.19
  Bottom 0.406: IC5.19 142.24,22.84 140.97,24.11 135.89,24.11 R41.2
SCL
  Bottom 0.61: JP2.2 45.72,44.43 44.45,45.7 IC1.28
SCL1
  Bottom 0.61: JP6.2 99.06,44.43 97.79,45.7 IC3.28
SCL2
  Bottom 0.61: JP10.2 152.4,44.43 151.13,45.7 IC5.28
SDA
  Bottom 0.61: JP2.3 45.72,41.89 44.45,43.16 IC1.27
SDA1
  Bottom 0.61: JP6.3 99.06,41.89 97.79,43.16 IC3.27
SDA2
  Bottom 0.61: JP10.3 152.4,41.89 151.13,43.16 IC5.27

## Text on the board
Bottom: v1.0 | v1.0 | v1.0 | B-0040 | B-0040 | B-0040 | www.sakul.cz | www.sakul.cz | www.sakul.cz | CO2 meter | CO2 meter | CO2 meter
